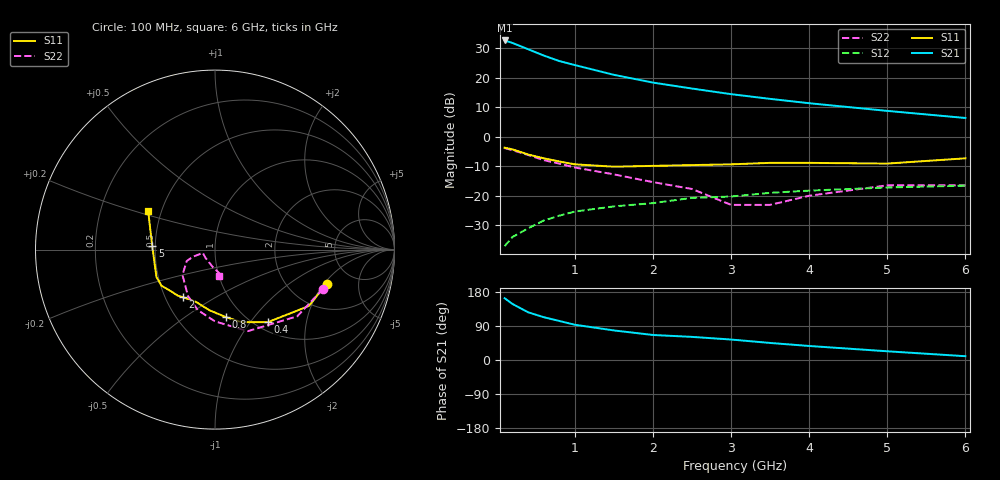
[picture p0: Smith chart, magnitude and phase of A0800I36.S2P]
!  MSA-0800 S AND NOISE PARAMETERS
!  Id=36mA  LAST UPDATED 07-27-92
# ghz s ma r 50
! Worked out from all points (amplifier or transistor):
!   14 points, 100 MHz to 6 GHz, reference 50 ohm
!   highest |S21| = 32.6 dB at 100 MHz (marker M1)
!   |S21| within 3 dB of that: start of sweep to 403.6 MHz
!   unconditionally stable (mu >= 1): 2.461 GHz to end of sweep
!   at 400 MHz: K = 0.64, MSG = 30.3 dB, |S12| = -31.1 dB
!   at 2 GHz: K = 0.97, MSG = 20.4 dB, |S12| = -22.5 dB
!   at 6 GHz: K = 1.39, MAG = 7.7 dB, |S12| = -16.6 dB
!   lowest NFmin = 2.40 dB at 100 MHz
!   S11 on the Smith chart (normalised r, x): 100 MHz: 3.22, -2.12; 400 MHz: 1.13, -1.22; 800 MHz: 0.83, -0.73; 2 GHz: 0.61, -0.36; 5 GHz: 0.48, +0.02; 6 GHz: 0.42, +0.22
0.1  0.65 -17.0  42.5 163.0  0.014 39.0  0.64 -20.0
0.2  0.61 -31.0  38.59 148.0  0.02 47.0  0.59 -39.0
0.4  0.5 -54.0  30.22 126.0  0.028 52.0  0.49 -68.0
0.6  0.43 -70.0  23.64 113.0  0.038 52.0  0.4 -90.0
0.8  0.38 -81.0  19.05 103.0  0.046 53.0  0.35 -106.0
1  0.34 -95.0  16.27 93.0  0.054 55.0  0.3 -120.0
1.5  0.31 -110.0  11.12 78.0  0.066 53.0  0.23 -142.0
2  0.32 -124.0  8.22 66.0  0.075 53.0  0.17 -158.0
2.5  0.33 -129.0  6.52 61.0  0.092 57.0  0.13 -162.0
3  0.34 -138.0  5.24 54.0  0.097 54.0  0.07 -165.0
3.5  0.36 -146.0  4.36 45.0  0.112 50.0  0.07 -140.0
4  0.36 -155.0  3.68 37.0  0.122 49.0  0.1 -96.0
5  0.35 177.0  2.73 23.0  0.138 43.0  0.15 -75.0
6  0.43 150.0  2.07 10.0  0.148 35.0  0.15 -81.0
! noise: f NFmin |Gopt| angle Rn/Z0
0.1  2.4  0.36  1  0.62
0.5  2.5  0.35  2  0.62
1  2.7  0.33  4  0.63
2  3.4  0.23  6  0.62
